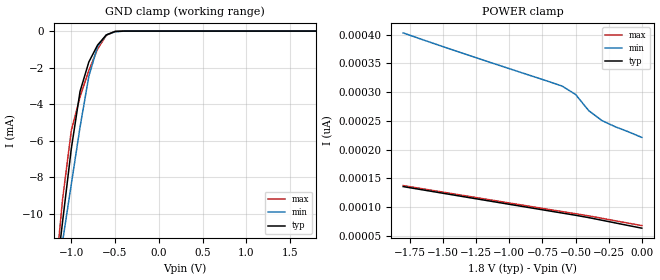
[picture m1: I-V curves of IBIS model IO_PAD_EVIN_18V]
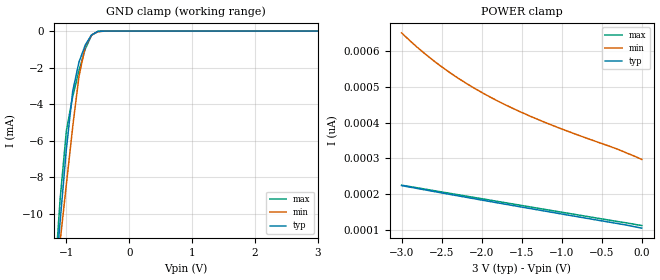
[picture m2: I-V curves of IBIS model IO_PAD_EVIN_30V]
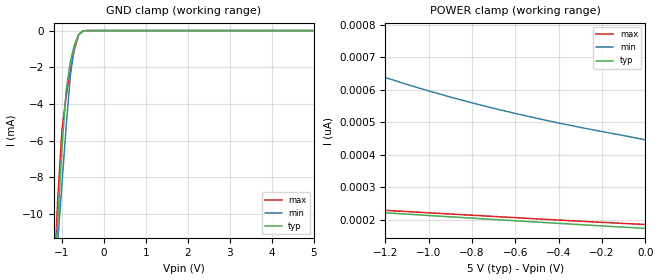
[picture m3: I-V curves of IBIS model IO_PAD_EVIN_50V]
[IBIS Ver]   3.2
[Comment Char]   |_char
[File name]   rx8901.ibs
[File Rev]   1.0
[Date]   2021/12/13 13:50:18
[Source]
[Notes]
[Disclaimer]
This information is for modeling purposes only, and is not guaranteed.
Property of SEIKO EPSON Corp.,
unauthorized reproduction and/or distribution is strictly prohibited.
[Copyright]
Copyright 2021, SEIKO EPSON Corp.
[Component]   rx8901
Si_location Pin
Timing_location Pin
[Manufacturer]   SEIKO EPSON Corp.
| PKG
[Package]
R_pkg   267m   NA   NA
L_pkg   2.8nH   NA   NA
C_pkg   0.70pF   NA   NA
[Pin] signal_name   model_name
1   VDD   POWER
2   VOUT   POWER
3   VBAT   POWER
4   FOUT   IO_PAD_FOUT_select
5   SCL   IO_PAD_SCL_select
6   EVIN1   IO_PAD_EVIN_select
7   SDA   IO_PAD_SDA_select
8   /INT   IO_PAD_XINT_select
9   GND   GND
10   EVIN2   IO_PAD_EVIN_select
[Model Selector]  IO_PAD_EVIN_select
IO_PAD_EVIN_18V   18V mode
IO_PAD_EVIN_30V   30V mode
IO_PAD_EVIN_50V   50V mode
[Model Selector]  IO_PAD_FOUT_select
IO_PAD_FOUT_18V   18V mode
IO_PAD_FOUT_30V   30V mode
IO_PAD_FOUT_50V   50V mode
[Model Selector]  IO_PAD_SCL_select
IO_PAD_SCL_18V   18V mode
IO_PAD_SCL_30V   30V mode
IO_PAD_SCL_50V   50V mode
[Model Selector]  IO_PAD_SDA_select
IO_PAD_SDA_18V   18V mode
IO_PAD_SDA_30V   30V mode
IO_PAD_SDA_50V   50V mode
[Model Selector]  IO_PAD_XINT_select
IO_PAD_XINT_18V   18V mode
IO_PAD_XINT_30V   30V mode
IO_PAD_XINT_50V   50V mode
| Models and submodels in the file (15): IO_PAD_EVIN_18V (Input), IO_PAD_EVIN_30V (Input), IO_PAD_EVIN_50V (Input), IO_PAD_FOUT_18V (3-state), IO_PAD_FOUT_30V (3-state), IO_PAD_FOUT_50V (3-state), IO_PAD_SCL_18V (Input), IO_PAD_SCL_30V (Input), IO_PAD_SCL_50V (Input), IO_PAD_SDA_18V (I/O_open_drain), IO_PAD_SDA_30V (I/O_open_drain), IO_PAD_SDA_50V (I/O_open_drain), IO_PAD_XINT_18V (Open_drain), IO_PAD_XINT_30V (Open_drain), IO_PAD_XINT_50V (Open_drain)
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[Model]   IO_PAD_EVIN_18V
Model_type Input
Polarity Non-Inverting
Vinh=1.26
Vinl=0.54
C_comp   2.5p   2.0p   3.0p
[Temperature Range] 25   105   -40
[Voltage Range]   1.80   1.60   2.00
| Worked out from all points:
|   GND clamp passes 1 mA (typ) near -0.73 V on its own axis
[GND Clamp]
-1.8V     -39.21mA   -33.96mA   -45.41mA
-1.2V     -14.49mA   -14.68mA   -14.3mA
-1.1V     -10.44mA   -11.52mA   -9.205mA
-1V       -6.43mA    -8.372mA   -5.441mA
-900mV    -3.296mA   -5.245mA   -3.59mA
-800mV    -1.693mA   -2.476mA   -2.16mA
-700mV    -766.3uA   -837.8uA   -984.2uA
-600mV    -208.2uA   -213.9uA   -229.3uA
-500mV    -22.05uA   -35.59uA   -13.65uA
-400mV    -1.255uA   -4.035uA   -297.2nA
1.8V      63.52pA    239.9pA    59.8pA
[POWER Clamp]
-1.8V     135.8pA    403.2pA    137.5pA
-1.4V     120.4pA    371.5pA    122.4pA
-600mV    89.77pA    310.6pA    92.33pA
-500mV    85.96pA    296.1pA    88.61pA
-400mV    81.84pA    267.9pA    84.89pA
-300mV    77.25pA    250.6pA    80.69pA
-200mV    72.62pA    239.9pA    76.32pA
0V        63.52pA    221.3pA    68.01pA
[Model]   IO_PAD_EVIN_30V
Model_type Input
Polarity Non-Inverting
Vinh=2.10
Vinl=0.90
C_comp   2.5p   2.0p   3.0p
[Temperature Range] 25   105   -40
[Voltage Range]   3.00   2.70   3.30
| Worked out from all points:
|   GND clamp passes 1 mA (typ) near -0.73 V on its own axis
[GND Clamp]
-3V       -89.62mA   -73.48mA   -108.8mA
-1.2V     -14.49mA   -14.68mA   -14.3mA
-1.1V     -10.44mA   -11.52mA   -9.208mA
-1V       -6.435mA   -8.376mA   -5.445mA
-900mV    -3.301mA   -5.25mA    -3.591mA
-800mV    -1.695mA   -2.481mA   -2.16mA
-700mV    -766.4uA   -841uA     -984.2uA
-600mV    -208.2uA   -214.1uA   -229.3uA
-500mV    -22.05uA   -35.6uA    -13.65uA
-300mV    -50.65nA   -360.3nA   -4.112nA
3V        105pA      325.8pA    99.83pA
[POWER Clamp]
-3V       224.2pA    651.5pA    225.4pA
-2.8V     215.9pA    610.3pA    217.8pA
-2.5V     203.7pA    556.7pA    206.4pA
-2.2V     191.7pA    511.4pA    195pA
-1.9V     179.8pA    472.7pA    183.7pA
-1.6V     168pA      439.1pA    172.3pA
-1.3V     156.3pA    409.5pA    161pA
-900mV    140.8pA    374.2pA    145.9pA
-300mV    117.9pA    325.8pA    123.6pA
0V        105pA      297.4pA    112.2pA
[Model]   IO_PAD_EVIN_50V
Model_type Input
Polarity Non-Inverting
Vinh=3.50
Vinl=1.50
C_comp   2.5p   2.0p   3.0p
[Temperature Range] 25   105   -40
[Voltage Range]   5.00   4.50   5.50
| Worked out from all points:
|   GND clamp passes 1 mA (typ) near -0.73 V on its own axis
[GND Clamp]
-5V       -176mA     -141.3mA   -217.5mA
-1.2V     -14.5mA    -14.69mA   -14.3mA
-1.1V     -10.44mA   -11.53mA   -9.209mA
-1V       -6.438mA   -8.379mA   -5.446mA
-900mV    -3.304mA   -5.253mA   -3.592mA
-800mV    -1.696mA   -2.485mA   -2.16mA
-700mV    -766.4uA   -843.3uA   -984.2uA
-600mV    -208.2uA   -214.2uA   -229.3uA
-500mV    -22.05uA   -35.6uA    -13.65uA
-300mV    -50.68nA   -360.3nA   -4.141nA
5V        173.9pA    512.6pA    165.8pA
[POWER Clamp]
-5V       420.9pA    3.125nA    380.9pA
-4.4V     380.7pA    2.419nA    352.8pA
-3.6V     334.3pA    1.704nA    320.9pA
-2.8V     293.5pA    1.2nA      290.2pA
-1.8V     247.6pA    794.3pA    252.2pA
-1.7V     243.2pA    764.5pA    248.4pA
-1.5V     234.6pA    709.7pA    240.9pA
-1.3V     226.1pA    660.8pA    233.3pA
-1.1V     217.8pA    617.2pA    225.7pA
-900mV    209.5pA    578.3pA    218.2pA
-500mV    193.3pA    512.6pA    203.2pA
0V        173.9pA    446.5pA    185.9pA
